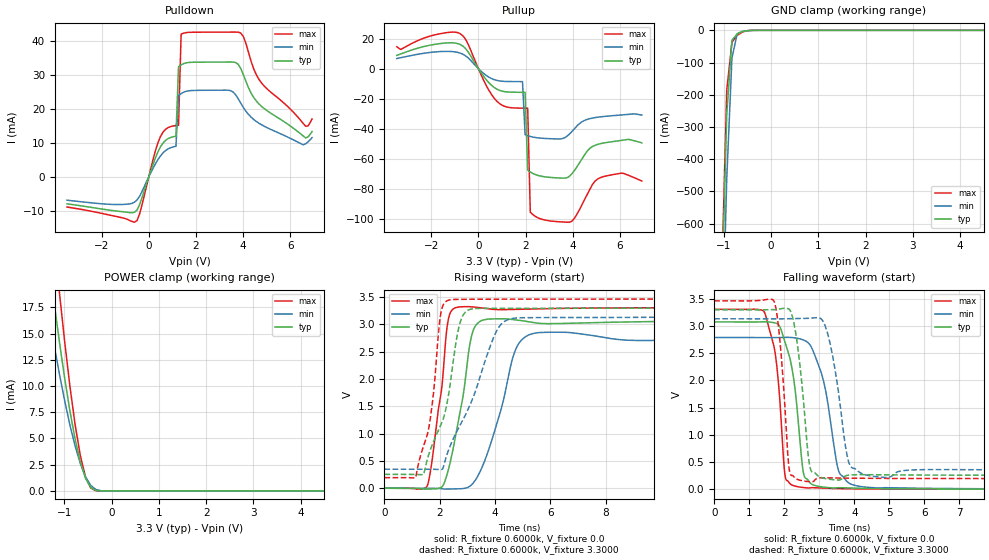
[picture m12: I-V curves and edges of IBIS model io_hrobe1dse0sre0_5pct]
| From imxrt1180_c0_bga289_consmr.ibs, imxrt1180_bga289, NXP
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[Model]  io_hrobe1dse0sre0_5pct
|   Model io_hrobe1dse0sre0_5pct
| This model was characterised for following simulation conditions:
| External (pad) voltage:
|   - Typ: 3.3V,   - Min: 3.135V,   - Max: 3.465V
| Library cells for typ/min/max conditions are connected as defined below:
|  PAD_IO - External Pad
|  ipp_do - Core Input
|  ipp_obe - Output Buffer Enable
|  ASRCN3V3[3] - NC
|  ASRCN3V3[4] - NC
|  ASRCP3V3[4] - NC
|  REFAPBIAS3V3 - gnde
|  REFBAMPL3V3 - vdd1v8
|  REFCAMPH3V3 - vdd1v8
|  REFDNBIAS3V3 - vdd1v8
|  REFH3V3 - REFH3V3
|  REFL3V3 - REFL3V3
|  gnde - gnde
|  ipp_dse - gnde
|  ipp_ina235_3v - NC
|  ipp_ina40_3v - NC
|  ipp_ina_mux - NC
|  ipp_ind - NC
|  ipp_ind_1p8v - NC
|  ipp_ind_3v - NC
|  ipp_sre - gnde
|  vdd - vdd
|  vdd1v8 - vdd1v8
|  vdda - vdde3v3
|  vdde3v3 - vdde3v3
| All other pins connected to ground
Model_type I/O
Polarity   Non-Inverting
Enable   Active-High
Vinl =   0.9900V
Vinh =   2.3100V
Vmeas =  1.6500V
Cref =   15.0000pF
Rref =   0.6000k
Vref =   0.0V
C_comp   4.0008pF   3.8187pF   4.1208pF
|C_comp_pullup   0.5645pF   0.7326pF   0.4701pF
|C_comp_pulldown   2.1156pF   2.2155pF   1.8988pF
[Model Spec]
| variable   typ   min   max
Vinh   2.3100V   NA   NA
Vinl   0.9900V   NA   NA
Vref   0.0V   0.0V   0.0V
Cref   15.0000pF   15.0000pF   15.0000pF
Rref   0.6000k   0.6000k   0.6000k
[Receiver Thresholds]
Vcross_high  =   0.0V
Vcross_low  =   0.0V
Vdiff_ac  =   0.0V
Vdiff_dc  =   0.0V
Tdiffslew_ac  =   0.0S
[Temperature Range]   25.0000   0.1250k   -40.0000
[Voltage Range]   3.3000V   3.1350V   3.4650V
[Pullup Reference]   3.3000V   3.1350V   3.4650V
[Pulldown Reference]   0.0V   0.0V   0.0V
[POWER Clamp Reference]   3.3000V   3.1350V   3.4650V
[GND Clamp Reference]   0.0V   0.0V   0.0V
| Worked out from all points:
|   slope of the pulldown table from 0 to 0.495 V, typ, clamps not added: 56 ohm
|   slope of the pullup table from 0 to 0.495 V, typ, clamps not added: 48.9 ohm
|   GND clamp passes 1 mA (typ) near -0.50 V on its own axis
|   POWER clamp passes 1 mA (typ) near -0.52 V on its own axis
|   rising waveform, R_fixture 0.6000k, V_fixture 0.0: 20-80 % time 596ps typ, 893ps min, 440ps max; typ from 0 V to 3.08 V
|   rising waveform, R_fixture 0.6000k, V_fixture 3.3000: 20-80 % time 811ps typ, 1.32ns min, 480ps max; typ from 0.254 V to 3.3 V
|   falling waveform, R_fixture 0.6000k, V_fixture 0.0: 20-80 % time 347ps typ, 470ps min, 268ps max; typ from 3.08 V to 0 V
|   falling waveform, R_fixture 0.6000k, V_fixture 3.3000: 20-80 % time 278ps typ, 378ps min, 215ps max; typ from 3.3 V to 0.254 V
[Pulldown]
|Voltage   I(typ)   I(min)   I(max)
-3.465V   -7.89mA    -6.82mA    -8.84mA
-495mV    -9.702mA   -6.763mA   -12.83mA
495mV     8.835mA    6.188mA    11.88mA
1.155V    12.02mA    9.055mA    15.17mA
1.265V    32.48mA    24mA       15.25mA
1.375V    33.05mA    24.59mA    42.1mA
1.485V    33.41mA    25mA       42.39mA
3.465V    33.87mA    25.46mA    42.69mA
3.905V    31.99mA    21.75mA    42.42mA
4.785V    20.82mA    15.41mA    27.71mA
6.655V    11.52mA    9.773mA    14.95mA
6.93V     13.4mA     11.6mA     17.1mA
[Pullup]
|Voltage   I(typ)   I(min)   I(max)
-3.465V   8.87mA     6.769mA    14.67mA
-770mV    16.12mA    10.37mA    23.31mA
660mV     -12.4mA    -7.253mA   -19.48mA
1.87V     -15.75mA   -8.628mA   -26.3mA
1.98V     -15.77mA   -43.96mA   -26.32mA
2.09V     -67.56mA   -44.66mA   -26.35mA
2.2V      -68.82mA   -45.19mA   -95.65mA
2.42V     -70.58mA   -45.87mA   -98.47mA
3.96V     -70.13mA   -42mA      -101.7mA
4.73V     -53mA      -33.27mA   -80.3mA
5.28V     -49.62mA   -31.91mA   -72.04mA
6.93V     -49.42mA   -30.89mA   -74.82mA
[GND_clamp]
|Voltage   I(typ)   I(min)   I(max)
-3.465V   -18.65A    -18.54A    -19.59A
-1.045V   -856.4mA   -1.07A     -789.2mA
-935mV    -262.9mA   -462.2mA   -186.4mA
-825mV    -31.14mA   -87.01mA   -37.16mA
-715mV    -11.21mA   -10.51mA   -15.88mA
-605mV    -3.859mA   -3.519mA   -5.394mA
-385mV    -79.74uA   -219.6uA   -43.96uA
6.93V     0A         0A         0A
[POWER_clamp]
|Voltage   I(typ)   I(min)   I(max)
-3.465V   98.76mA    78.08mA    125.9mA
-1.43V    25.63mA    19.65mA    34.12mA
-1.32V    21.65mA    16.67mA    28.86mA
-1.21V    17.8mA     13.81mA    23.74mA
-1.1V     14.15mA    11.1mA     18.82mA
-880mV    7.624mA    6.286mA    9.977mA
-770mV    4.936mA    4.278mA    6.317mA
-660mV    2.762mA    2.615mA    3.373mA
-550mV    1.207mA    1.351mA    1.33mA
-440mV    332.8uA    528.9uA    282.4uA
-330mV    37.59uA    131uA      15.04uA
6.93V     0A         0A         0A
[Ramp]
| variable   typ   min   max
dV/dt_r  1.8464/0.5956n   1.6742/0.8930n   1.9857/0.4397n
dV/dt_f  1.8274/0.2775n   1.6719/0.3778n   1.9622/0.2150n
R_load = 0.6000k
[Rising Waveform]
R_fixture= 0.6000k
V_fixture= 0.0
V_fixture_min= 0.0
V_fixture_max= 0.0
|time   V(typ)   V(min)   V(max)
0s        180nV      2.99uV     125.3nV
1.557ns   -16.18mV   -575.6uV   57.42mV
2.058ns   17.05mV    -5.707mV   1.787V
2.293ns   308.7mV    -15.02mV   3.054V
2.724ns   1.381V     -10.39mV   3.322V
3.104ns   2.689V     44.43mV    3.325V
3.341ns   3.009V     193.3mV    3.313V
4.755ns   3.083V     2.557V     3.277V
5.557ns   3.023V     2.849V     3.287V
60ns      3.077V     2.79V      3.31V
[Rising Waveform]
R_fixture= 0.6000k
V_fixture= 3.3000
V_fixture_min= 3.1350
V_fixture_max= 3.4650
|time   V(typ)   V(min)   V(max)
0s        254.3mV    348.5mV    194.7mV
1.129ns   254mV      348.4mV    201.6mV
1.631ns   663.3mV    348.5mV    1.189V
2.047ns   1.167V     343.9mV    3.234V
2.443ns   2.164V     858.5mV    3.456V
2.702ns   2.978V     1.125V     3.459V
2.94ns    3.235V     1.356V     3.461V
4.046ns   3.295V     2.874V     3.461V
4.787ns   3.295V     3.119V     3.462V
60ns      3.3V       3.135V     3.465V
[Falling Waveform]
R_fixture= 0.6000k
V_fixture= 0.0
V_fixture_min= 0.0
V_fixture_max= 0.0
|time   V(typ)   V(min)   V(max)
0s        3.077V     2.79V      3.31V
1.416ns   3.08V      2.79V      3.273V
1.861ns   3.003V     2.789V     1.755V
2.045ns   2.654V     2.794V     185.5mV
2.534ns   350.7mV    2.748V     31.07mV
2.674ns   172.1mV    2.698V     21.05mV
3.124ns   37.04mV    1.98V      18.11mV
3.563ns   27.26mV    316.5mV    9.682mV
4.443ns   12.95mV    31.1mV     3.458mV
60ns      676.4nV    2.205uV    424.4nV
[Falling Waveform]
R_fixture= 0.6000k
V_fixture= 3.3000
V_fixture_min= 3.1350
V_fixture_max= 3.4650
|time   V(typ)   V(min)   V(max)
0s        3.3V       3.135V     3.465V
1.706ns   3.303V     3.135V     3.459V
1.877ns   3.316V     3.133V     2.73V
2.164ns   3.292V     3.136V     292.1mV
2.388ns   2.6V       3.137V     176.6mV
2.74ns    393.5mV    3.146V     134.7mV
3.241ns   187.2mV    2.858V     208mV
3.872ns   260.6mV    444.6mV    201.5mV
4.804ns   264.4mV    218.9mV    197.4mV
60ns      254.3mV    348.5mV    194.7mV
